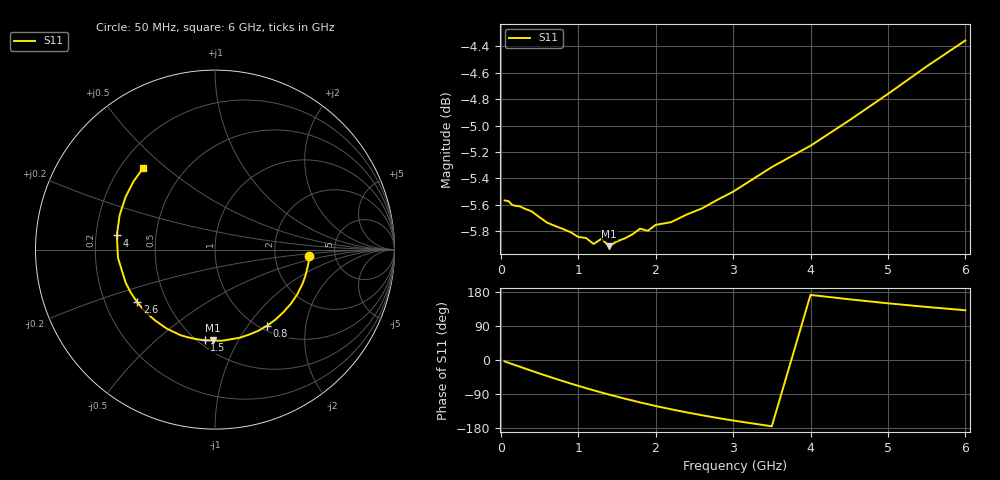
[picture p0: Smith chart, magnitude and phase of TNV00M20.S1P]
! SIEMENS Discrete & RF Semiconductors
! BAS70-07W
! Si Schottky Diode in SOT343
! IF = 0.2 mA
! S-Parameters:  February  1997
# GHz  S  MA  R  50
!  f  S11
! GHz  MAG  ANG
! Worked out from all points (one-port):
!   34 points, 50 MHz to 6 GHz, reference 50 ohm
!   lowest |S11| = -5.9 dB at 1.4 GHz (marker M1), VSWR 3.05, Z = 29.1 - j39.6 ohm
!   |S11| at or under -10 dB: nowhere
!   S11 on the Smith chart (normalised r, x): 50 MHz: 3.20, -0.30; 800 MHz: 1.08, -1.24; 1.5 GHz: 0.54, -0.73; 2.6 GHz: 0.34, -0.27; 4 GHz: 0.29, +0.07; 6 GHz: 0.29, +0.42
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0.05  0.5268 -3.7
0.1  0.5265 -7.4
0.25  0.5241 -18.0
0.4  0.5218 -28.6
0.5  0.5192 -35.6
0.6  0.5167 -42.4
0.7  0.5153 -49.0
0.8  0.5139 -55.5
0.9  0.5125 -62.0
1.1  0.5099 -74.2
1.2  0.5072 -80.0
1.3  0.5095 -85.8
1.4  0.5062 -91.3
1.5  0.5084 -96.6
1.6  0.5097 -102.0
1.8  0.514 -112.0
2  0.5157 -121.4
2.2  0.517 -130.0
2.4  0.5204 -138.2
2.6  0.5232 -145.8
2.8  0.5272 -153.0
3  0.5308 -159.7
3.5  0.5424 -175.0
4  0.5526 171.8
4.5  0.5649 160.2
5  0.5781 149.6
5.5  0.5921 140.0
6  0.6057 131.2
